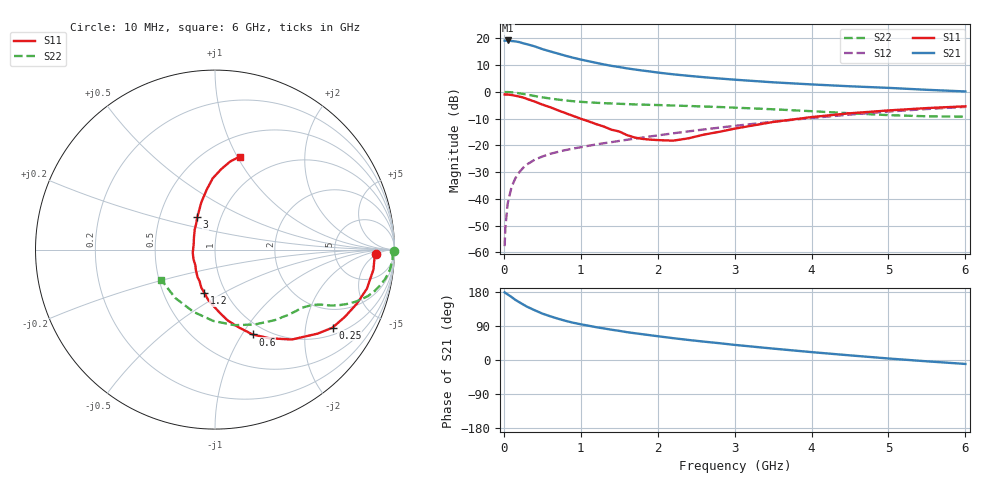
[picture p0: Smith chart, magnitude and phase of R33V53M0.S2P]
! SIEMENS Small Signal Semiconductors
! BFR181
! Si NPN RF Bipolar Junction Transistor in SOT23
! VCE = 3.5 V  IC = 3 mA
! Common Emitter S-Parameters:  May  1996
# GHz  S  MA  R  50
!  f  S11  S21  S12  S22
! GHz  MAG  ANG  MAG  ANG  MAG  ANG  MAG  ANG
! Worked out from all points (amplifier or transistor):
!   36 points, 10 MHz to 6 GHz, reference 50 ohm
!   highest |S21| = 19.2 dB at 50 MHz (marker M1)
!   |S21| within 3 dB of that: start of sweep to 477.8 MHz
!   unconditionally stable (mu >= 1): 1.371 GHz to 3.18 GHz
!   at 250 MHz: K = 0.30, MSG = 23.3 dB, |S12| = -28.4 dB
!   at 1.4 GHz: K = 1.01, MAG = 13.7 dB, |S12| = -18.8 dB
!   at 6 GHz: K = 0.86, MSG = 2.9 dB, |S12| = -5.6 dB
!   lowest NFmin = 1.40 dB at 450 MHz
!   S11 on the Smith chart (normalised r, x): 10 MHz: 17, -5; 250 MHz: 1.24, -2.82; 600 MHz: 0.86, -1.11; 1.2 GHz: 0.80, -0.41; 3 GHz: 0.77, +0.29; 6 GHz: 0.70, +1.02
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0.01  0.8963 -1.7  9.053 178.6  0.0013 91.2  0.9959 -0.6
0.02  0.89 -2.9  9.034 177.0  0.0029 90.7  0.9895 -1.4
0.05  0.8897 -7.2  9.145 173.0  0.0082 85.3  0.9906 -3.3
0.15  0.8458 -20.9  8.788 158.6  0.0243 77.5  0.9623 -9.8
0.2  0.8151 -27.3  8.522 152.6  0.0312 75.2  0.9392 -12.4
0.25  0.786 -33.6  8.107 146.6  0.0379 71.6  0.9156 -14.9
0.3  0.7381 -39.4  7.78 140.8  0.0439 69.2  0.8894 -17.0
0.4  0.6588 -49.5  7.095 131.4  0.0537 64.9  0.8363 -20.3
0.5  0.5792 -58.5  6.307 122.5  0.0617 62.3  0.7891 -22.7
0.6  0.5172 -66.1  5.72 115.6  0.0693 60.3  0.7516 -24.4
0.7  0.4533 -73.0  5.218 109.2  0.0751 59.1  0.7184 -25.7
0.8  0.4014 -79.8  4.741 103.5  0.0813 58.1  0.6911 -26.6
0.9  0.3545 -85.5  4.349 98.4  0.087 58.0  0.6686 -27.3
1.1  0.2811 -98.0  3.743 90.5  0.098 58.2  0.6367 -28.9
1.2  0.2493 -103.6  3.49 86.6  0.1038 58.3  0.6249 -29.7
1.6  0.1555 -133.2  2.749 73.5  0.1269 59.0  0.5905 -32.9
2.2  0.1222 166.7  2.129 57.6  0.1676 59.6  0.5551 -39.6
3  0.205 118.8  1.689 39.9  0.2311 56.9  0.5064 -51.7
3.5  0.2732 106.3  1.508 30.1  0.2762 53.7  0.472 -62.1
4.5  0.3977 91.8  1.271 12.2  0.3759 44.5  0.3977 -91.3
5.5  0.4973 80.3  1.092 -3.5  0.4774 32.0  0.3488 -129.5
6  0.5365 75.1  1.017 -10.4  0.5232 24.8  0.3435 -150.4
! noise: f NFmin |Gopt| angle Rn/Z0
0.45  1.4  0.56  17  0.36
0.9  1.5  0.45  35  0.34
1.8  1.85  0.25  82  0.36
